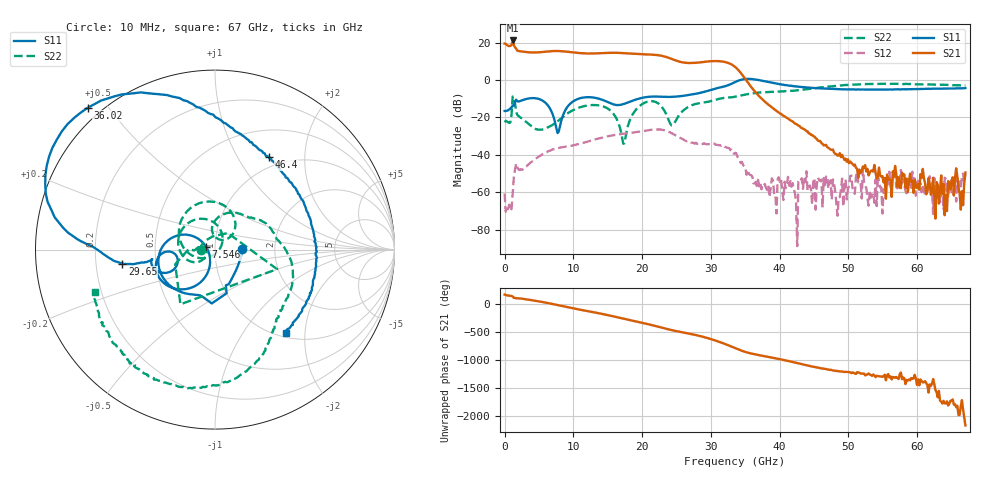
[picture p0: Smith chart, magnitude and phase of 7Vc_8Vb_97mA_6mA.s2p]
! MARKI MICROWAVE INC.
! Date:  05/05/2020
! Model Number:  APM-7099CH
! Description:  2-port Small Signal S-parameter data for APM-7099CH
! Frequency Range:  10 MHz to 67 GHz
! Port Configuration:  PORT 1: Input
!  PORT 2: Output
! Bias Condition: Vc = +7V, Vb = +8V
! APM-7099CH s2p files are only valid for small signal conditions (below -5 dBm input power)
!S2P File: Measurements: Mag<S11> Ang<S11>, Mag<S21> Ang<S21>, Mag<S12> Ang<S12>, Mag<S22> Ang<S22>!row 1
# Hz S  dB  R 50
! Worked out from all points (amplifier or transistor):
!   401 points, 10 MHz to 67 GHz, reference 50 ohm
!   highest |S21| = 21.2 dB at 1.182 GHz (marker M1)
!   |S21| within 3 dB of that: start of sweep to 653.5 MHz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
!   unconditionally stable (mu >= 1): start of sweep to 34.09 GHz; 36.98 GHz to end of sweep
!   at 11.06 GHz: K = 4.13, MAG = 15.1 dB, |S12| = -33.9 dB
!   at 33.51 GHz: K = 3.60, MAG = 14.5 dB, |S12| = -38.9 dB
!   at 67 GHz: K = 14656.01, MAG = -44.4 dB, |S12| = -50.0 dB
!   S11 on the Smith chart (normalised r, x): 10 MHz: 1.35, +0.01; 7.546 GHz: 0.91, +0.02; 29.65 GHz: 0.32, -0.07; 36.02 GHz: -0.04, +0.45; 46.4 GHz: 0.86, +1.37; 67 GHz: 1.09, -1.60
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1e7  -16.53 0.9  19.50 178.5  -60.64 109.1  -22.47 -178.7
1.182325e9  -13.69 -68.1  21.17 143.1  -60.87 74.7  -8.81 -17.5
1.68475e9  -10.44 -93.4  16.80 111.1  -44.64 -82.2  -16.68 178.9
4.866775e9  -9.98 -172.3  14.82 58.1  -41.26 -176.6  -26.52 -178.1
7.546375e9  -25.95 164.5  15.54 -7.4  -36.58 117.5  -22.53 -141.8
9.3886e9  -13.22 -116.7  15.03 -56.0  -35.27 78.8  -17.27 -149.1
1.123082e10  -9.48 -144.3  14.34 -100.0  -33.73 45.2  -14.26 -176.1
1.47478e10  -11.34 -177.6  14.49 175.0  -30.25 -27.8  -14.70 111.2
1.759488e10  -12.44 -156.0  14.35 96.7  -28.53 -94.6  -30.30 -102.9
2.027448e10  -9.30 -159.5  13.76 22.4  -27.23 -159.6  -12.29 143.4
2.245165e10  -8.85 -169.8  13.22 -43.9  -26.40 135.8  -12.76 67.3
2.379145e10  -9.00 -171.4  11.97 -87.0  -27.54 91.2  -20.75 40.8
2.580115e10  -8.51 -170.1  9.52 -140.2  -31.40 39.9  -16.89 94.5
2.797832e10  -7.21 -170.0  9.27 164.6  -34.03 3.4  -12.66 61.1
2.965308e10  -5.64 -171.5  9.98 109.8  -34.17 -30.9  -11.57 42.4
3.183025e10  -3.53 179.4  9.81 19.1  -34.95 -94.2  -9.58 20.8
3.3505e10  -1.09 170.2  7.05 -65.3  -38.91 -165.4  -8.89 7.7
3.601712e10  0.52 131.9  -4.44 -167.5  -51.52 66.9  -7.12 -12.2
4.472582e10  -4.15 68.8  -29.33 -36.9  -66.55 35.9  -4.59 -59.2
4.640058e10  -4.48 59.6  -34.93 -75.3  -52.41 -101.4  -3.72 -66.7
5.594665e10  -5.04 6.4  -52.69 125.7  -48.97 -129.9  -2.02 -115.5
6.7e10  -4.28 -49.4  -49.45 -18.3  -50.03 58.0  -2.98 -160.4
